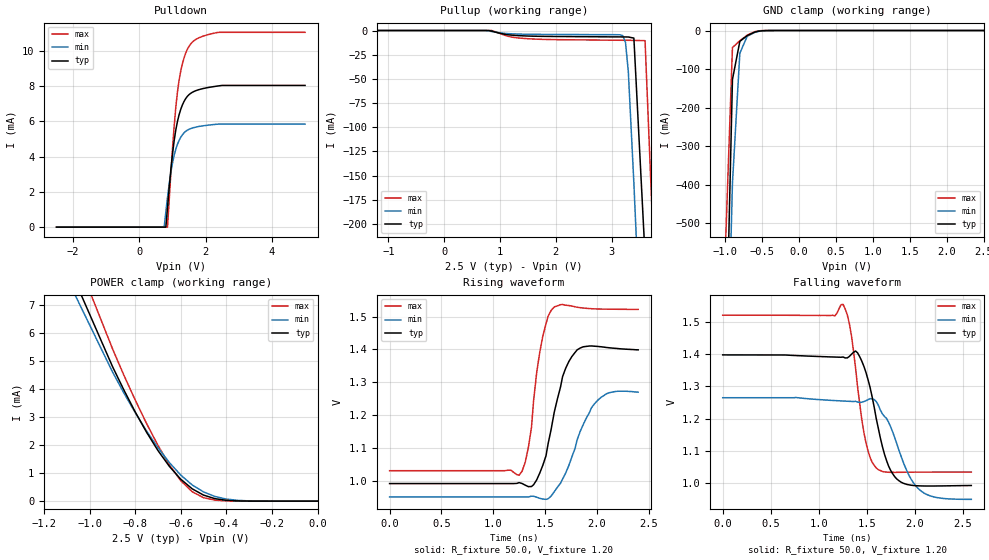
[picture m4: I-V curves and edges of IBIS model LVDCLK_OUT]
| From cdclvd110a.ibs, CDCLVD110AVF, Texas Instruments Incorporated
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|   LVD110 Output  MODEL
[Model]   LVDCLK_OUT
Model_type   Output
Polarity   Non-Inverting
| Signals   Q0_T,Q0_N,Q1_T,Q1_N,Q2_T,Q2_N,Q3_T,Q3_N,Q4_T,Q4_N,Q5_T,Q5_N,
|   Q6_T,Q6_N,Q7_T,Q7_N,Q8_T,Q8_N,Q9_T,Q9_N
Vmeas = 1.20V   |Reference voltage for timing measurements
Cref = 0pF   |Timing specification test load capacitance value
Rref = 50ohms   |Note: 50 Ohm load; single ended configuration
Vref = 1.20V   |Timing specification test load voltage
| variable   typ   min   max
C_comp   3.3pF   3.2pF   3.4pF
|   typ   min   max
[Temperature Range]   50   105   -40
[Voltage range]   2.5V   2.375V   2.625V
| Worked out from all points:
|   GND clamp passes 1 mA (typ) near -0.51 V on its own axis
|   POWER clamp passes 1 mA (typ) near -0.62 V on its own axis
|   rising waveform, R_fixture 50.0, V_fixture 1.20: 20-80 % time 164ps typ, 241ps min, 116ps max; typ from 0.991 V to 1.4 V
|   falling waveform, R_fixture 50.0, V_fixture 1.20: 20-80 % time 185ps typ, 260ps min, 132ps max; typ from 1.4 V to 0.992 V
[Pulldown]
|   Voltage   I(typ)   I(min)   I(max)
-2.5V     -29.62nA   -23.25nA   -36.44nA
750mV     168.4pA    548.4nA    25.78pA
800mV     15.05nA    858.2uA    29.54pA
850mV     1.093mA    1.688mA    2.872nA
1V        4.131mA    3.631mA    4.447mA
1.1V      5.509mA    4.421mA    6.781mA
1.15V     5.993mA    4.698mA    7.659mA
1.3V      6.933mA    5.241mA    9.271mA
1.5V      7.514mA    5.549mA    10.26mA
1.8V      7.798mA    5.709mA    10.74mA
2.35V     7.999mA    5.838mA    11.04mA
5V        8.038mA    5.842mA    11.05mA
[Pullup]
|   Voltage   I(typ)   I(min)   I(max)
| Note that the[Pullup]voltage table is referenced to Vcc
| and is calculated using Vtable=Vcc - Vmeasured.
-2.5V     21.51nA    18.28nA    27.74nA
750mV     74.65pA    -465.2pA   8.821pA
850mV     -601uA     -1.001mA   -48.6pA
1.15V     -4.413mA   -3.22mA    -6.028mA
1.45V     -5.596mA   -3.817mA   -8.266mA
3.2V      -6.619mA   -5.167mA   -10.08mA
3.25V     -6.651mA   -12.34mA   -10.09mA
3.3V      -6.695mA   -42.26mA   -10.11mA
3.4V      -7.829mA   -157.8mA   -10.21mA
3.6V      -232.7mA   -418.5mA   -10.49mA
3.8V      -572.4mA   -680mA     -292.8mA
5V        -2.612A    -2.249A    -2.945A
[GND_clamp]
|   Voltage   I(typ)   I(min)   I(max)
| Outputs in High Impedance (off)
-2.5V     -15.78A    -12.64A    -19.33A
-1.1V     -1.777A    -1.871A    -1.136A
-900mV    -127mA     -396.1mA   -44.29mA
-800mV    -28.2mA    -58.96mA   -26.37mA
-700mV    -13.08mA   -14.74mA   -12.13mA
-600mV    -4.294mA   -4.917mA   -2.982mA
-400mV    -51.17uA   -111.5uA   -6.838uA
2.5V      438.5pA    53.68nA    76.12pA
[POWER_clamp]
|   Voltage   I(typ)   I(min)   I(max)
| Note that the [POWER_clamp] voltage table is referenced to Vcc
| and is calculated using Vtable = Vcc - Vmeasured.
| Outputs in Tri-state.
-2.5V     39.25mA    38.42mA    36.89mA
-1.1V     8.539mA    7.97mA     9.556mA
-900mV    4.815mA    4.621mA    5.452mA
-800mV    3.188mA    3.161mA    3.614mA
-700mV    1.806mA    1.907mA    1.99mA
-650mV    1.242mA    1.378mA    1.296mA
-600mV    782.8uA    930uA      730.7uA
-550mV    440.2uA    578.5uA    337.2uA
-500mV    215.1uA    328uA      122.8uA
-400mV    29.86uA    73.51uA    8.503uA
-300mV    1.969uA    8.472uA    398.9nA
0V        438.5pA    3.262nA    198.5pA
[Ramp]
|   typ   min   max
dV/dt_r   0.2395V/0.171ns   0.1841V/0.230ns   0.2835V/0.118ns
dV/dt_f   0.2367V/0.184ns   0.1801V/0.250ns   0.2811V/0.131ns
R_load = 50   | Note: The measurement is single-ended with 50ohm
|   to Vref.
[Rising Waveform]
R_fixture = 50.0
V_fixture = 1.20
V_fixture_min = 1.11
V_fixture_max = 1.28
|   time   V(typ)   V(min)   V(max)
0s        990.8mV    950mV      1.03V
1.25ns    993.7mV    950mV      1.016V
1.34ns    981.4mV    950.1mV    1.101V
1.42ns    1.002V     949.2mV    1.33V
1.48ns    1.047V     943.4mV    1.442V
1.56ns    1.157V     952.8mV    1.519V
1.67ns    1.317V     1.005V     1.537V
1.81ns    1.399V     1.123V     1.529V
2.04ns    1.408V     1.253V     1.523V
2.4ns     1.399V     1.27V      1.522V
[Falling Waveform]
R_fixture = 50.0
V_fixture = 1.20
V_fixture_min = 1.11
V_fixture_max = 1.28
|   time   V(typ)   V(min)   V(max)
0s        1.398V     1.265V     1.522V
1.255ns   1.392V     1.255V     1.555V
1.341ns   1.4V       1.253V     1.459V
1.427ns   1.393V     1.25V      1.247V
1.513ns   1.322V     1.259V     1.1V
1.599ns   1.201V     1.253V     1.046V
1.707ns   1.069V     1.2V       1.033V
1.836ns   1.006V     1.101V     1.033V
2.095ns   990mV      968.4mV    1.033V
2.59ns    991.5mV    948.4mV    1.033V
